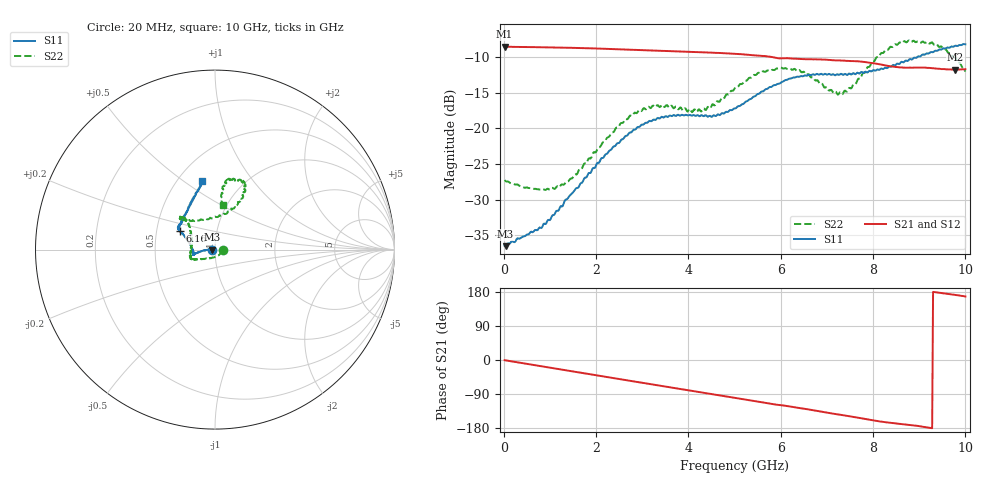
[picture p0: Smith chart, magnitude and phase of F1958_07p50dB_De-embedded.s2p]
! Integrated Device Technology
! Corporate Headquarters
! 6024 Silver Creek Valley Road
! San Jose, CA 95138  USA
! Phone:  1-408-284-8200
! Toll Free:  1-800-223-1366
! Webpage:  http://www.idt.com/
! Timing and RF Division
! 515 Groton Road, Suite 102
! Westford, MA 01886-6024
! Device:  F1958
! Description: 7-bit 0.25 dB Digital Step Attenuator
! Frequency:  0.001 -  6.000 GHz
! Package:  4x4 mm Thin QFN Plastic Package: 24 pin
! Ports:  2 RF, 12 DC
!  Pin  1  = D0
!  Pin  2  = VDD
!  Pin  3  = VMODE
!  Pin  4  = GND
!  Pin  5  = RF1  =  Port 1
!  Pin  6  = GND
!  Pin  7  = GND
!  Pin  8  = GND
!  Pin  9  = GND
!  Pin 10  = GND
!  Pin 11  = GND
!  Pin 12  = GND
!  Pin 13  = GND
!  Pin 14  = RF2  =  Port 2
!  Pin 15  = GND
!  Pin 16  = LE
!  Pin 17  = CLK
!  Pin 18  = DATA
!  Pin 19  = D6
!  Pin 20  = D5
!  Pin 21  = D4
!  Pin 22  = D3
!  Pin 23  = D2
!  Pin 24  = D1
! State:  30
! Atten State:  7.50 dB
! Voltage:  +3.30 Volts
! Current:  0.258 mA
! Data:  The device was measured on a F1958 evaluation board which has
!  individual transmission lines to the RF pins.  Data was collected
!  using a calibrated network analyzer.  The evaluation board was
!  de-embedded using Automatic Fixture Removal (AFR).
!  The reference plane is the edge of the package pin.
! Misc:
!  Action Tracker AT0419
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# GHz S dB R 50
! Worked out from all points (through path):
!   500 points, 20 MHz to 10 GHz, reference 50 ohm
!   highest |S21| = -8.49 dB at 20 MHz (marker M1); lowest = -11.7 dB at 9.78 GHz (marker M2)
!   group delay of S21, straight-line fit = 54 ps
!   lowest |S11| = -36.5 dB at 40 MHz (marker M3), VSWR 1.03, Z = 48.5 - j0.0843 ohm
!   |S11| at or under -10 dB: start of sweep to 8.95 GHz
!   |S22| runs from -28.6 to -7.6 dB; largest |S21 - S12| = 0.0012
!   S11 on the Smith chart (normalised r, x): 20 MHz: 0.97, -0.00; 6.16 GHz: 0.66, +0.14; 10 GHz: 0.65, +0.59
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0.02  -36.48 -176.8  -8.49 -0.6  -8.48 -0.5  -27.27 -3.6
0.04  -36.55 -176.7  -8.50 -1.0  -8.49 -0.9  -27.40 -5.4
0.78  -33.92 176.6  -8.58 -15.8  -8.58 -15.8  -28.59 -45.1
1.08  -32.17 179.5  -8.61 -21.8  -8.60 -21.8  -28.44 -67.5
1.44  -29.38 -179.0  -8.66 -29.1  -8.65 -29.1  -27.10 -99.0
1.7  -27.61 -177.1  -8.70 -34.2  -8.70 -34.1  -25.57 -117.7
2.62  -21.18 -171.7  -8.89 -52.5  -8.88 -52.5  -18.81 -151.5
2.98  -19.50 -169.5  -8.98 -59.7  -8.97 -59.8  -17.56 -155.8
3.36  -18.58 -167.1  -9.07 -67.2  -9.08 -67.3  -16.87 -159.8
4.3  -18.15 -171.2  -9.27 -85.8  -9.28 -85.8  -17.42 165.4
5.02  -17.18 169.7  -9.50 -100.1  -9.51 -100.1  -14.23 138.1
5.54  -15.08 157.9  -9.77 -110.4  -9.77 -110.4  -12.19 134.5
6.16  -13.08 152.1  -10.13 -122.0  -10.14 -122.0  -11.66 137.4
6.68  -12.42 149.2  -10.27 -132.0  -10.29 -131.9  -12.79 133.7
7.1  -12.46 145.5  -10.39 -140.9  -10.40 -140.8  -14.59 115.0
7.36  -12.47 143.3  -10.46 -146.0  -10.47 -145.9  -14.95 91.2
7.92  -11.90 133.2  -10.73 -157.7  -10.73 -157.7  -11.34 65.0
8.34  -11.32 123.7  -11.22 -165.3  -11.23 -165.3  -8.81 62.5
8.74  -10.52 115.8  -11.46 -170.4  -11.47 -170.4  -7.83 67.0
9.24  -9.29 106.1  -11.51 -179.3  -11.51 -179.4  -8.03 77.4
9.78  -8.37 101.3  -11.73 171.7  -11.75 171.7  -10.02 82.8
10  -8.17 100.8  -11.66 167.6  -11.70 167.7  -11.99 80.3
